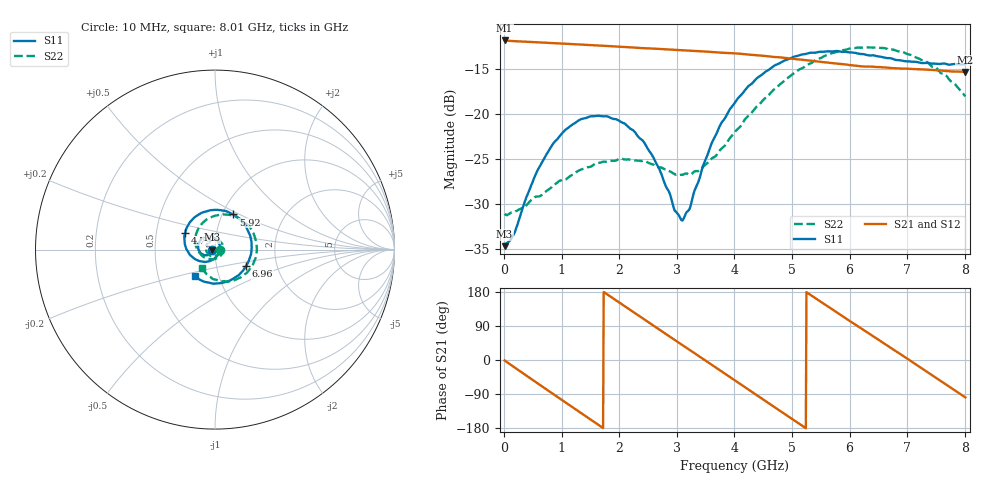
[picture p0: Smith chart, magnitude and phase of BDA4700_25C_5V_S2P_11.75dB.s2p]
!Agilent Technologies,E5071B,MY42404982,A.09.10
!Date: Mon Oct 20 13:31:59 2025
!Data & Calibration Information:
!Freq	S11:SOLT2(ON)	S21:SOLT2(ON)	S12:SOLT2(ON)	S22:SOLT2(ON)
# Hz S RI R 50
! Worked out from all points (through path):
!   801 points, 10 MHz to 8.01 GHz, reference 50 ohm
!   highest |S21| = -11.86 dB at 10 MHz (marker M1); lowest = -15.4 dB at 8 GHz (marker M2)
!   group delay of S21, straight-line fit = 283 ps
!   lowest |S11| = -34.7 dB at 10 MHz (marker M3), VSWR 1.04, Z = 48.2 - j0.0994 ohm
!   |S11| at or under -10 dB: start of sweep to end of sweep
!   |S22| runs from -31.3 to -12.6 dB; largest |S21 - S12| = 0.0018
!   S11 on the Smith chart (normalised r, x): 10 MHz: 0.96, -0.00; 4.79 GHz: 0.70, +0.14; 5.92 GHz: 1.13, +0.46; 6.96 GHz: 1.39, -0.27; 8.01 GHz: 0.76, -0.24
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1e7  -0.0183 -0.00103  0.2551 -0.00552  0.2552 -0.00585  0.0277 -0.00144
1.6e8  -0.019 -0.00901  0.2416 -0.0749  0.2416 -0.0749  0.0268 -0.00898
7.2e8  -0.0486 -0.0315  0.0605 -0.2403  0.0605 -0.2404  -0.000704 -0.0367
1.02e9  -0.0751 -0.0231  -0.0719 -0.2344  -0.0719 -0.2344  -0.0267 -0.0333
1.35e9  -0.0933 0.00479  -0.1887 -0.1513  -0.1888 -0.1515  -0.0483 -0.0081
1.93e9  -0.068 0.0638  -0.2203 0.0853  -0.2204 0.0854  -0.0278 0.0471
2.41e9  -0.0115 0.0697  -0.0773 0.218  -0.0774 0.2182  0.0235 0.0493
2.68e9  0.0149 0.048  0.0319 0.2268  0.0319 0.2266  0.0431 0.026
2.97e9  0.0266 0.0107  0.138 0.179  0.1381 0.1787  0.0455 -0.00619
3.11e9  0.0243 -0.0087  0.1773 0.1385  0.1769 0.1387  0.04 -0.0223
3.54e9  -0.0159 -0.0577  0.2198 -0.0226  0.2197 -0.0229  -0.00417 -0.0533
4.01e9  -0.0994 -0.0586  0.1272 -0.1749  0.1272 -0.1746  -0.0705 -0.0355
4.39e9  -0.1573 -0.00199  -0.0111 -0.2109  -0.011 -0.2113  -0.1073 0.0226
4.79e9  -0.1659 0.0943  -0.1429 -0.1475  -0.1425 -0.1481  -0.0975 0.1078
5.35e9  -0.0674 0.2074  -0.1928 0.0382  -0.193 0.0377  0.0156 0.1916
5.92e9  0.1021 0.1958  -0.0677 0.1751  -0.0681 0.1749  0.1716 0.1473
6.31e9  0.182 0.1075  0.0542 0.1745  0.0548 0.1737  0.2295 0.0433
6.68e9  0.2033 -0.00959  0.1464 0.1043  0.1468 0.1043  0.2181 -0.0662
6.96e9  0.1727 -0.0921  0.1763 0.0238  0.1761 0.023  0.1719 -0.1329
7.49e9  0.0377 -0.1857  0.1212 -0.1255  0.1209 -0.1256  0.0326 -0.1785
8e9  -0.1117 -0.1508  -0.0232 -0.169  -0.0233 -0.1693  -0.0712 -0.1037
8.01e9  -0.1141 -0.1492  -0.0261 -0.1686  -0.0261 -0.1688  -0.0724 -0.1015
